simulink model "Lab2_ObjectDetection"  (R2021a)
settings: Solver=ode4  StartTime=0.0  StopTime=inf  FixedStep=1/30  RelTol=1e-3  EnableMultiTasking=on
undefined symbols (not defined in the file): directions, height, HxWx3, imread, intmax, left, MATLAB, N, NE, NW, qc_get_step_size, RGB, S, SE, SW, top, Video3D, W, width, x
libraries: quarc_library x20, simulink x1

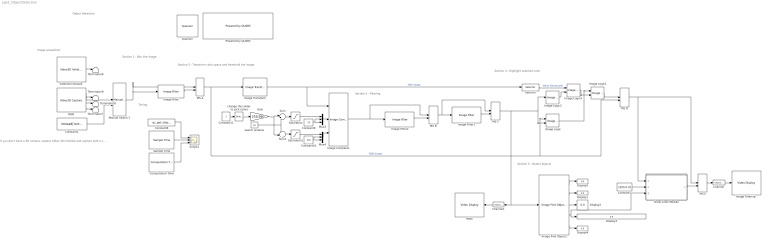
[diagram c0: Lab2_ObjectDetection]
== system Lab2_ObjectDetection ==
  note: Section 4 - Highlight selected color
  note: Section 3 - Filtering
  note: Section 2 - Transform color space and threshold the image
  note: Section 1 - Blur the image
  note: Timing
  note: Object Detection
  note: Section 5 - Detect objects
  note: Image acquisition
  note: If you don't have a 3D camera, replace Video 3D initialize and capture with a video capture block. Manual switches will allow you to visualize the image and the mask as filters are applied based on the color selected in Section 2. The last switch allows you to visualize the color of interest with a box bounding the biggest object in that color.
  Channel : quarc_library/Signal Routing/Channel  channel=0  buffer_size=1
  Channel1 : quarc_library/Signal Routing/Channel  channel=1  buffer_size=1
  Computation Time : quarc_library/Sources/Time/Computation Time  sample_time=qc_get_step_size  use_model=on  use_cpu_time=off
  Constant1 : Constant  Value=imread('octopus.jpg');
  Constant10 : Constant  Value=255
  Constant11 : Constant
  Constant7 : Constant  Value=[255 0 0]
  Constant8 : Constant  Value=qc_get_step_size
  Constant9 : Constant  Value=25
  Display{1..5} (5 alike) : Display
  Draw Lines Module : MATLAB Function  TreatAsAtomicUnit=on
  Gain : Gain  Gain=255/360
  Image Compare1 : quarc_library/Image Processing/Generic/Image Compare  output_type=Combined (one HxW output)  source=External input ports  r_comparison=min <= pixel and pixel <= max with wrapping  r_minimum=0  r_maximum=10  g_comparison=min <= pixel and pixel <= max with wrapping  g_minimum=0  g_maximum=64  b_comparison=min <= pixel and pixel <= max with wrapping  b_minimum=0  b_maximum=200
  Image Filter : quarc_library/Image Processing/Generic/Image Filter  filter_type=Gaussian  source_of_roi=Internal dialog parameter  roi_style=[top, left, height, width]  roi=[]  maximum_roi=[]  roi_zone=Operate inside region of interest  border_type=Replicate  border_value=[0 0 0]  kernel_size=5  sigma=1  mask_size=[3 3]  kernel=int16([-2 -1 0; -1 1 1; 0 1 2])  divisor=1  offset=0  rounding=Nearest  algorithm_hint=None  threshold=100  alpha=0.9  num_frames=8  num_valid=1  gap_threshold=10  depth_threshold=255  iterations=2
  Image Filter1 : quarc_library/Image Processing/Generic/Image Filter  filter_type=Maximum  source_of_roi=Internal dialog parameter  roi_style=[top, left, height, width]  roi=[]  maximum_roi=[]  roi_zone=Operate inside region of interest  border_type=Replicate  border_value=[0 0 0]  kernel_size=15  sigma=.2  mask_size=[5 5]  kernel=int16([-2 -1 0; -1 1 1; 0 1 2])  divisor=1  offset=0  rounding=Nearest  algorithm_hint=None  threshold=100  alpha=0.9  num_frames=8  num_valid=1  gap_threshold=10  depth_threshold=255  iterations=2
  Image Filter2 : quarc_library/Image Processing/Generic/Image Filter  filter_type=Minimum  source_of_roi=Internal dialog parameter  roi_style=[top, left, height, width]  roi=[]  maximum_roi=[]  roi_zone=Operate inside region of interest  border_type=Replicate  border_value=[0 0 0]  kernel_size=15  sigma=.2  mask_size=[5 5]  kernel=int16([-2 -1 0; -1 1 1; 0 1 2])  divisor=1  offset=0  rounding=Nearest  algorithm_hint=None  threshold=100  alpha=0.9  num_frames=8  num_valid=1  gap_threshold=10  depth_threshold=255  iterations=2
  "Image Filtering " : quarc_library/Multimedia/Video Display  Tag=Lab2_ObjectDetection/Image Filtering  sample_time=-1  use_hardware=on
  Image Find Objects : quarc_library/Image Processing/Generic/Image Find Objects  num_objects=1  connectivity=8 directions (N, NE, E, SE, S, SW, W, NW)  sort_order=Sort by number of pixels  min_pixels=10  max_pixels=intmax('uint32')  largest=on  exclude_at_edges=off  variable_size=off  use_complex=off
  Image Logic : quarc_library/Image Processing/Generic/Image Logic  algorithm=AND  source=Internal dialog parameter  row=0  column=0
  Image Logic1 : quarc_library/Image Processing/Generic/Image Logic  algorithm=OR  source=Internal dialog parameter  row=0  column=0
  Image Logic2 : quarc_library/Image Processing/Generic/Image Logic  algorithm=NOT  source=Internal dialog parameter  row=0  column=0
  Image Logic4 : quarc_library/Image Processing/Generic/Image Logic  algorithm=AND  source=Internal dialog parameter  row=0  column=0
  Image Transform : quarc_library/Image Processing/Generic/Image Transform  algorithm=RGB to HSV  color_theme=KRYGCBMW  min_pixel=0  max_pixel=4000  focal_length=308  principal_point=[262 334]  radial_coeffs=[-0.3129 0.0907]  tangential_coeffs=[]  extrapolated_pixel=0  interpolation=nearest  row_coords=0  column_coords=0  output_height=480  output_width=640  angle=0  origin=[240 320]  output_origin=[240 320]  output_data_type=uint8
  MS A : ManualSwitch  CurrentSetting=0
  MS B : ManualSwitch  CurrentSetting=0
  MS C : ManualSwitch  CurrentSetting=0
  MS D : ManualSwitch
  MS E : ManualSwitch  CurrentSetting=0
  Manual Switch 1 : ManualSwitch
  Mask : quarc_library/Multimedia/Video Display  Tag=Lab2_ObjectDetection/Mask  sample_time=-1  use_hardware=on
  Mux3 : Mux  Inputs=3
  Mux4 : Mux  Inputs=3
  Powered by QUARC : quarc_library/Logos/Powered by QUARC
  Quanser : quarc_library/Logos/Quanser
  RGB : quarc_library/Multimedia/Video3D Capture  object_name=Video3D-1  stream_type=RGB  stream_index=0  resolution=640 x 480  width=640  height=480  output_format=MATLAB RGB (HxWx3)  data_type=uint8  sample_time=qc_get_step_size  camera_intrinsics=off  depth_scale=off  brightness_override=off  brightness=50.0  contrast_override=off  contrast=50.0  hue_override=off  hue=50.0  saturation_override=off  saturation=50.0  sharpness_override=off  sharpness=50.0  gamma_override=off  gamma=50.0  gain_override=off  gain=50.0  backlightcompensation_override=off  backlightcompensation=50.0  whitebalance_override=Automatic white balance  whitebalance=50.0  exposure_override=Automatic exposure  exposure=30.0  emitter=Enable laser emitter  preset=Do not set camera presets
  Sample Time : quarc_library/Sources/Time/Sample Time  Priority=-99  sample_time=qc_get_step_size
  Saturation : Saturate  UpperLimit=255  LowerLimit=0
  Saturation1 : Saturate  UpperLimit=255  LowerLimit=0
  Scope1 : Scope  NumInputPorts=3
  Selector : Selector  NumberOfDimensions=3  InputPortWidth=3  IndexOptions=Select all,Select all,Index vector (dialog)  Indices=[1 3],1,3  OutputSizes=1,1,1
  Sum : Sum  Inputs=|+-
  Sum1 : Sum  Inputs=++|
  Terminator{6..9} (4 alike) : Terminator
  Video3D Initialize : quarc_library/Multimedia/Video3D Initialize  object_name=Video3D-1  source=Device  identifier=0  file=sample.bag  sample_time=qc_get_step_size  active=on
  change this slider to pick colors : simulink/Math Operations/Slider Gain  gain=180  low=0  high=360
  search window : Constant  Value=20
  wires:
  Sample Time/1 -> Scope1/2
  Image Compare1/1 -> MS B/1, Image Filter2/1
  Image Find Objects/1 -> Display5/1
  Image Find Objects/2 -> Display1/1
  Image Find Objects/3 -> Display2/1
  Image Find Objects/4 -> Draw Lines Module/3(pts), Display3/1
  Constant7/1 -> Draw Lines Module/2(color)
  Image Transform/1 -> Selector/1, Image Compare1/1  "HSV Image"
  Image Find Objects/5 -> Display4/1
  Image Filter1/1 -> MS C/2
  MS D/1 -> Draw Lines Module/1(img_in), MS E/1
  Constant8/1 -> Scope1/1
  Computation Time/1 -> Scope1/3
  Mux3/1 -> Image Compare1/2
  Mux4/1 -> Image Compare1/3
  Sum1/1 -> Saturation1/1
  Saturation1/1 -> Mux4/1
  Sum/1 -> Saturation/1
  Gain/1 -> Sum1/2, Sum/1
  change this slider to pick colors/1 -> Gain/1
  Constant9/1 -> Mux3/3, Mux3/2
  Saturation/1 -> Mux3/1
  Constant10/1 -> Mux4/2, Mux4/3
  Constant11/1 -> change this slider to pick colors/1
  Draw Lines Module/1(img_out) -> MS E/2
  Channel/1 -> "Image Filtering "/1
  MS E/1 -> Channel/1
  Image Logic1/1 -> MS D/1
  Channel1/1 -> Mask/1
  Image Filter2/1 -> MS B/2
  MS B/1 -> Image Filter1/1, MS C/1
  Selector/1 -> Image Logic4/1  "Value (Greyscale)"
  Image Logic/1 -> Image Logic1/1
  MS A/1 -> Image Logic/1, MS D/2, Image Transform/1  "RGB Image"
  Image Logic2/1 -> Image Logic4/2
  search window/1 -> Sum1/1, Sum/2
  MS C/1 -> Image Logic2/1, Image Logic/2, Image Find Objects/1, Channel1/1
  Image Logic4/1 -> Image Logic1/2
  Manual Switch 1/1 -> MS A/1, Image Filter/1
  Image Filter/1 -> MS A/2
  Constant1/1 -> Manual Switch 1/2
  RGB/2 -> Terminator9/1
  RGB/3 -> Terminator8/1
  RGB/4 -> Terminator7/1
  Video3D Initialize/1 -> Terminator6/1
  RGB/1 -> Manual Switch 1/1

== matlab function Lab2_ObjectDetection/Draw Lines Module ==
function img_out = drawLines(img_in, color, pts)

% Draw lines connecting the points using the provided color

% Inputs:
% img_in    : Input RGB Image (size = m by n)
% color     : 1x3 matrix of RGB color values for each marker
% pts       : p x-y pairs of points (px) where markers are to be drawn

% Outputs:
% img_out   : Output RGB Image with the markers drawn in (size = m by n)

%% Initialization
if size(img_in, 3) == 3
    img_out = img_in;
elseif size(img_in, 3) == 1
    img_out = cat(3, img_in, img_in, img_in);
end

box = single(pts (:,1)); % data on the box of the largest object

pts = [box(1), box(2); box(1), box(4); box(3), box(4); box(3), box(2); box(1), box(2)];

%points = pts;

[p, ~] = size(pts); % determine the number of points

%% Draw the lines

    for i = 1:p-1
        % determine the max(rows_difference, col_difference) between two
        % points
        itr = ceil(max(abs(pts(i,1) - pts(i+1,1)), abs(pts(i,2) - pts(i+1,2))));
        
        % generate linear spaces of row and col values between the pts
        row_vec = round(linspace(pts(i,1), pts(i+1,1), itr));
        col_vec = round(linspace(pts(i,2), pts(i+1,2), itr));
        
        % iterate through the values and shade them right

        for j = 1:itr
            img_out(row_vec(j), col_vec(j),1) = color(1);
            img_out(row_vec(j), col_vec(j),2) = color(2);
            img_out(row_vec(j), col_vec(j),3) = color(3);
        end
    end
end
